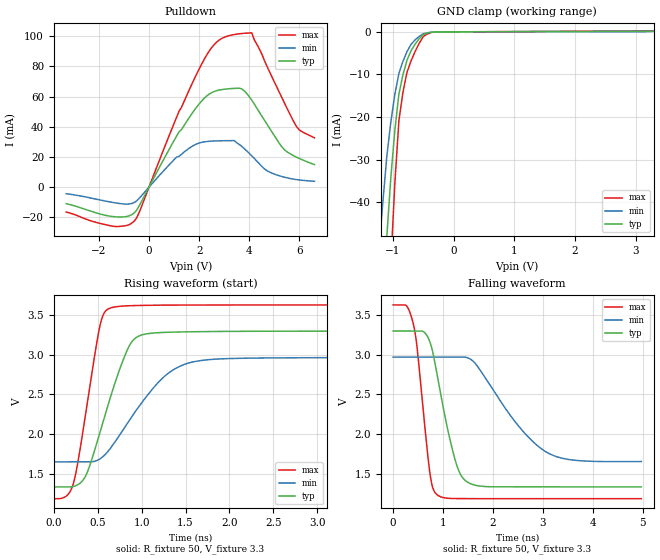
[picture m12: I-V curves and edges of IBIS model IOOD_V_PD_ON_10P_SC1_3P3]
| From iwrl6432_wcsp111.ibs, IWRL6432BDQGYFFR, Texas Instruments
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|   Model Cell IOOD_V_PD_ON_10P_SC1_3P3
|IOOD_V_PD_ON_10P_SC1_3P3
[Model]   IOOD_V_PD_ON_10P_SC1_3P3
Model_type   I/O_open_drain
Polarity   Non-Inverting
Enable   Active-Low
Vinl =  0.8V
Vinh =  2V
Cref =  15pF
Rref =  100.0000M
Vref =  0V
Vmeas =  1.65
|   typ   min   max
C_comp   2.059994p   1.912853p   2.135747p
[Model Spec]
Vinl   0.8V   0.8V   0.8V
Vinh   2V   2V   2V
[Temperature Range]   25   125   -40
[Voltage Range]   3.3   2.97   3.63
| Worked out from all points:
|   slope of the pulldown table from 0 to 0.495 V, typ, clamps not added: 31.8 ohm
|   GND clamp passes 1 mA (typ) near -0.52 V on its own axis
|   rising waveform, R_fixture 50, V_fixture 3.3: 20-80 % time 334ps typ, 532ps min, 208ps max; typ from 1.33 V to 3.3 V
|   falling waveform, R_fixture 50, V_fixture 3.3: 20-80 % time 385ps typ, 931ps min, 233ps max; typ from 3.3 V to 1.33 V
| Where Nom  PVT is Nominal Process, 3.3V, 25C
|   Fast PVT is Strong Process,  3.63V, -40C
|   Slow PVT is Weak Process,   2.97V, 125C
[Pulldown]
|   voltage   I(typ)   I(min)   I(max)
-3.3V     -10.93mA   -4.311mA   -16.48mA
-1.4V     -19.53mA   -10.23mA   -25.96mA
-600mV    -17.23mA   -10.26mA   -22.66mA
1.1V      33.82mA    19.89mA    46.25mA
2V        55.14mA    29.24mA    78.29mA
2.6V      63.35mA    30.61mA    94.44mA
3.2V      65.21mA    30.81mA    100.4mA
3.7V      65.09mA    27.02mA    101.8mA
4.1V      57.64mA    20.71mA    102.2mA
5.3V      26.68mA    7.058mA    59.31mA
5.9V      19.77mA    5.007mA    39.76mA
6.6V      14.97mA    3.923mA    32.7mA
[GND_clamp]
|   voltage   I(typ)   I(min)   I(max)
-3.3V     -787.2mA   -607.8mA   -1.235A
-1.233V   -85.66mA   -52.14mA   -138.8mA
-1.167V   -66.47mA   -40.37mA   -107.7mA
-1.1V     -48.25mA   -29.37mA   -77.99mA
-1.033V   -34.28mA   -21.19mA   -54.56mA
-966.7mV  -23.07mA   -14.67mA   -35.51mA
-900mV    -14.62mA   -9.792mA   -20.84mA
-833.3mV  -10.07mA   -6.938mA   -14.17mA
-700mV    -4.435mA   -2.939mA   -6.836mA
-500mV    -641.2uA   -454.5uA   -1.12mA
-300mV    -31.62uA   -32.73uA   -44.27uA
3.3V      108.6uA    159.4uA    198.5uA
[Ramp]
| variable   typ   min   max
dV/dt_f  1.1800539/0.38506764n 0.79469436/0.93858809n  1.4663953/0.23379182n
dV/dt_r  1.1731734/0.46682563n 0.80227934/1.080283n   1.4754285/0.24457461n
R_load = 50
[Rising Waveform]
R_fixture = 50
V_fixture = 3.3
V_fixture_min = 2.97
V_fixture_max = 3.63
|   time   V(typ)   V(min)   V(max)
0s        1.335V     1.651V     1.187V
223.4ps   1.341V     1.651V     1.381V
365.8ps   1.482V     1.651V     2.282V
518.6ps   1.998V     1.684V     3.33V
630.3ps   2.415V     1.802V     3.582V
810.3ps   2.992V     2.09V      3.614V
921.6ps   3.202V     2.274V     3.619V
1.262ns   3.281V     2.729V     3.624V
1.555ns   3.289V     2.902V     3.625V
4.974ns   3.298V     2.966V     3.627V
[Falling Waveform]
R_fixture = 50
V_fixture = 3.3
V_fixture_min = 2.97
V_fixture_max = 3.63
|   time   V(typ)   V(min)   V(max)
0s        3.298V     2.969V     3.626V
269.8ps   3.298V     2.969V     3.614V
406.5ps   3.298V     2.969V     3.383V
483ps     3.298V     2.969V     3.075V
735.8ps   3.162V     2.969V     1.517V
887.5ps   2.728V     2.969V     1.233V
1.253ns   1.652V     2.969V     1.188V
1.512ns   1.388V     2.956V     1.187V
3.068ns   1.335V     1.774V     1.186V
4.974ns   1.334V     1.654V     1.186V
